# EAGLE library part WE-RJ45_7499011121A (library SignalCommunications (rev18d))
Order Code 7499011121A Design THT xBase-T 10/100 Base-T Ports 1x1 Application Standard Tab Position DOWN LED (Left-Right) Yellow-Green EMI Fingers Yes Details see: http://katalog.we-online.de/en/pbs/WE-LAN_RJ45/7499011121A? Updated by Yingchun Shan 2016-08-29 2016(C) Würth Elektronik
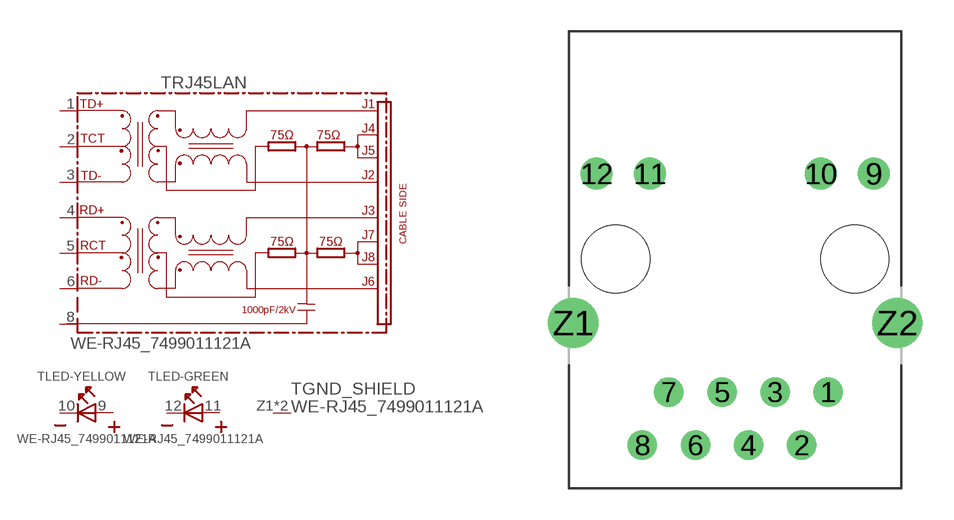
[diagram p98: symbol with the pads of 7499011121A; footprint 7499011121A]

Designator prefix T; gates RJ45LAN=74990X-THT-10/100-T LED-YELLOW=LED2PIN LED-GREEN=LED2PIN GND_SHIELD=GND_PIN

## WE-RJ45_7499011121A (COMPANY-URL: http://www.we-online.de; CREATED-BY: Christin Zierenner; CREATED-DATE: AUG 2012; DATASHEET-URL: http://katalog.we-online.de/kataloge/eisos/media/pdf/7499011121A.pdf; MANUFACTURER: Würth Elektronik eiSos GmbH)  [7499011121A]
1  RJ45LAN:TD+
2  RJ45LAN:TCT
3  RJ45LAN:TD-
4  RJ45LAN:RD+
5  RJ45LAN:RCT
6  RJ45LAN:RD-
8  RJ45LAN:8
9  LED-YELLOW:A  pas
10  LED-YELLOW:K  pas
11  LED-GREEN:A  pas
12  LED-GREEN:K  pas
Z1  GND_SHIELD:1  pwr
Z2  GND_SHIELD:1  pwr

## Footprint 7499011121A (pad centres in mm)
MAX HEIGHT=13.90mm PORTS----1X1 LED --YES
drill 0.9: 1 4.445,-6.35; 2 3.175,-8.89; 3 1.905,-6.35; 4 0.635,-8.89; 5 -0.635,-6.35; 6 -1.905,-8.89; 7 -3.175,-6.35; 8 -4.445,-8.89
drill 1.02: 9 6.63,4.08; 10 4.09,4.08; 11 -4.09,4.08; 12 -6.63,4.08
drill 1.6: Z1 -7.745,-3.05; Z2 7.745,-3.05
hole 3.25 at 5.715,0
hole 3.25 at -5.715,0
